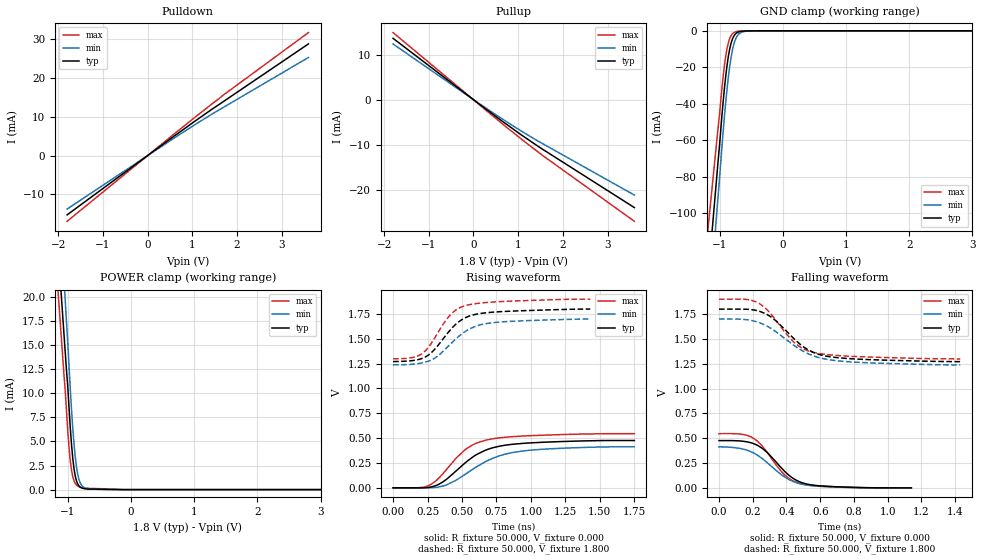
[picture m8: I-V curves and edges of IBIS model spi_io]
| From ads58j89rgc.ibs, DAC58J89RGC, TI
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[Model]   spi_io
Model_type I/O
Vinl=4.000E-01
Vinh=1.200E+00
Vref=0.000E+00
Rref=1.000E+06
Cref=0.000E+00
Vmeas=9.000E-01
C_comp   5.590E-13   4.480E-13   6.700E-13
[Voltage Range]   1.800E+00   1.700E+00   1.900E+00
[POWER Clamp Reference]   1.800E+00   1.700E+00   1.900E+00
[GND Clamp Reference]   0.000E+00   0.000E+00   0.000E+00
[Pullup Reference]   1.800E+00   1.700E+00   1.900E+00
[Pulldown Reference]   0.000E+00   0.000E+00   0.000E+00
[Temperature Range]   25   85   -40
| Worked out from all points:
|   slope of the pulldown table from 0 to 0.27 V, typ, clamps not added: 118 ohm
|   slope of the pullup table from 0 to 0.27 V, typ, clamps not added: 133 ohm
|   GND clamp passes 1 mA (typ) near -0.72 V on its own axis
|   POWER clamp passes 1 mA (typ) near -0.86 V on its own axis
|   rising waveform, R_fixture 50.000, V_fixture 0.000: 20-80 % time 279ps typ, 328ps min, 244ps max; typ from 0 V to 0.476 V
|   falling waveform, R_fixture 50.000, V_fixture 0.000: 20-80 % time 171ps typ, 190ps min, 157ps max; typ from 0.476 V to 0 V
|   rising waveform, R_fixture 50.000, V_fixture 1.800: 20-80 % time 211ps typ, 240ps min, 187ps max; typ from 1.27 V to 1.8 V
|   falling waveform, R_fixture 50.000, V_fixture 1.800: 20-80 % time 215ps typ, 251ps min, 188ps max; typ from 1.8 V to 1.27 V
[GND Clamp]
-1.8V     -385.2mA   -432mA     -322.5mA
-1.02V    -70.49mA   -89.56mA   -52.24mA
-940mV    -37.9mA    -54.21mA   -24.11mA
-900mV    -24.26mA   -38.47mA   -13.41mA
-880mV    -18.67mA   -31.54mA   -9.48mA
-840mV    -10.1mA    -19.83mA   -4.312mA
-800mV    -4.874mA   -11.28mA   -1.809mA
-760mV    -2.19mA    -5.833mA   -740.3uA
-720mV    -960.5uA   -2.826mA   -303.2uA
-680mV    -430.3uA   -1.348mA   -133.7uA
-520mV    -46.51uA   -97.78uA   -40.34uA
3.6V      0A         0A         0A
[Power Clamp]
-1.8V     86.4mA     105.5mA    80.49mA
-1.06V    16.24mA    21.98mA    11.99mA
-1.04V    14.34mA    19.73mA    10.37mA
-1V       10.78mA    15.36mA    6.162mA
-960mV    6.496mA    10.53mA    3.019mA
-940mV    4.688mA    8.325mA    2.033mA
-900mV    2.152mA    4.7mA      907.9uA
-840mV    561.9uA    1.538mA    364.9uA
-800mV    253uA      664.5uA    244.6uA
-740mV    97.31uA    214.7uA    166.3uA
-480mV    42.11uA    15.46uA    97.8uA
3.6V      0A         0A         0A
[Pullup]
-1.8V     13.6mA     12.35mA    14.88mA
120mV     -913.1uA   -819uA     -1.017mA
960mV     -7.028mA   -6.285mA   -7.853mA
1.64V     -11.58mA   -10.26mA   -13.04mA
3.6V      -23.93mA   -21.16mA   -26.97mA
[Pulldown]
-1.8V     -15.26mA   -13.76mA   -16.92mA
600mV     5.079mA    4.568mA    5.642mA
1.7V      13.95mA    12.45mA    15.67mA
3.6V      28.78mA    25.28mA    31.69mA
[Rising Waveform]
R_fixture = 50.000
V_fixture = 0.000
V_fixture_min = 0.000
V_fixture_max = 0.000
|  time   V(typ)   V(min)   V(max)
0s        0V         0V         0V
200ps     -486.7uV   -418.7uV   2.659mV
270ps     6.758mV    377uV      30.27mV
370ps     67.51mV    21.3mV     155.4mV
520ps     247.6mV    133.1mV    380.1mV
590ps     321mV      197.6mV    440.8mV
680ps     383.7mV    269.8mV    482.1mV
810ps     428.1mV    337.5mV    508.7mV
980ps     450.9mV    376.6mV    524mV
1.75ns    476.1mV    413.1mV    545.3mV
[Falling Waveform]
R_fixture = 50.000
V_fixture = 0.000
V_fixture_min = 0.000
V_fixture_max = 0.000
|  time   V(typ)   V(min)   V(max)
0s        476.1mV    413.1mV    545.3mV
130ps     471.5mV    395.5mV    540.9mV
200ps     448.7mV    355.7mV    503.8mV
230ps     426.4mV    326.7mV    466.6mV
280ps     365.2mV    262.7mV    370.6mV
390ps     165.4mV    109mV      130.4mV
430ps     106.9mV    71.27mV    79.18mV
480ps     59.56mV    41.52mV    44.14mV
650ps     14.86mV    10.87mV    13.32mV
1.14ns    0V         0V         0V
[Rising Waveform]
R_fixture = 50.000
V_fixture = 1.800
V_fixture_min = 1.700
V_fixture_max = 1.900
|  time   V(typ)   V(min)   V(max)
0s        1.271V     1.238V     1.299V
140ps     1.281V     1.245V     1.312V
210ps     1.302V     1.258V     1.351V
280ps     1.364V     1.288V     1.46V
410ps     1.581V     1.439V     1.734V
460ps     1.653V     1.505V     1.795V
520ps     1.71V      1.571V     1.833V
620ps     1.752V     1.636V     1.858V
740ps     1.77V      1.665V     1.872V
1.43ns    1.8V       1.7V       1.9V
[Falling Waveform]
R_fixture = 50.000
V_fixture = 1.800
V_fixture_min = 1.700
V_fixture_max = 1.900
|  time   V(typ)   V(min)   V(max)
0s        1.8V       1.7V       1.9V
160ps     1.799V     1.694V     1.898V
240ps     1.779V     1.663V     1.855V
320ps     1.707V     1.593V     1.727V
440ps     1.509V     1.441V     1.474V
500ps     1.422V     1.375V     1.401V
560ps     1.364V     1.329V     1.364V
650ps     1.323V     1.291V     1.341V
780ps     1.301V     1.269V     1.325V
1.43ns    1.271V     1.238V     1.299V
[Ramp]
dV/dt_r   2.8599E-01/2.7828E-10   2.4805E-01/3.2723E-10   3.2658E-01/2.4320E-10
dV/dt_f   3.1727E-01/2.1387E-10   2.7715E-01/2.5127E-10   3.6076E-01/1.8780E-10
R_load = 50
